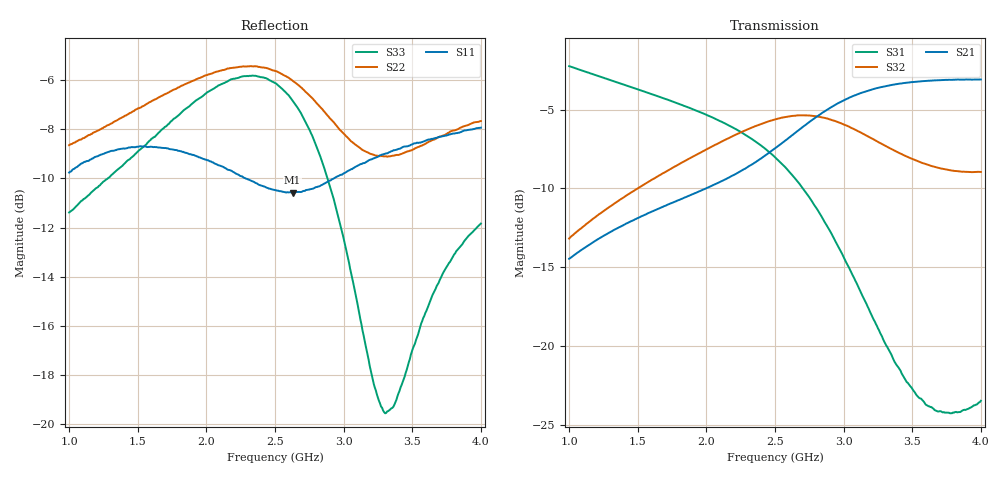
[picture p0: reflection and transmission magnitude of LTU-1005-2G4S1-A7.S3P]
!Agilent Technologies,E5071C,MY46104616,A.09.54
!Date: Mon Mar 28 16:57:22 2011
!Data & Calibration Information:
!Freq	S11:SOLT3(ON)	S12:SOLT3(ON)	S13:SOLT3(ON)
!	S21:SOLT3(ON)	S22:SOLT3(ON)	S23:SOLT3(ON)
!	S31:SOLT3(ON)	S32:SOLT3(ON)	S33:SOLT3(ON)
# Hz S dB R 50
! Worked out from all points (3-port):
!   401 points, 1 GHz to 4 GHz, reference 50 ohm
!   strongest paths, dB at 1 GHz, 1.75 GHz, 2.5 GHz, 3.25 GHz, 4 GHz:
!     S21: -14.5, -10.9, -7.5, -3.6, -3.1
!     S32: -13.2, -8.7, -5.6, -7.0, -9.0
!     S31: -2.2, -4.5, -8.0, -18.9, -23.5
!   lowest |S11| = -10.6 dB at 2.627 GHz (marker M1), VSWR 1.84, Z = 27.2 + j1.98 ohm
!   |S11| at or under -10 dB: 2.286 GHz to 2.929 GHz (643.1 MHz wide, 24.7 % of centre)
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1e9  -9.76 -148.9  -14.47 57.6  -2.24 -54.4
     -14.47 57.7  -8.65 114.4  -13.19 47.3
     -2.24 -54.4  -13.19 47.2  -11.38 -179.4
1.4425e9  -8.75 -167.1  -12.14 48.7  -3.54 -75.4
          -12.12 48.6  -7.34 86.8  -10.33 27.9
          -3.54 -75.4  -10.32 27.7  -9.22 131.3
1.915e9  -9.07 -179.9  -10.32 42.8  -5.02 -100.8
         -10.31 42.7  -6.01 58.3  -7.93 2.8
         -5.03 -100.8  -7.93 2.8  -6.87 78.3
2.1925e9  -9.73 175.5  -9.17 41.0  -6.14 -119.4
          -9.18 40.9  -5.50 41.3  -6.69 -15.9
          -6.14 -119.4  -6.68 -15.9  -5.95 47.4
2.5e9  -10.47 173.4  -7.46 38.5  -8.01 -144.8
       -7.47 38.4  -5.63 21.9  -5.63 -42.5
       -8.02 -144.8  -5.63 -42.5  -6.12 10.2
2.6275e9  -10.58 173.6  -6.60 36.2  -9.17 -156.8
          -6.61 36.2  -6.02 14.8  -5.39 -55.6
          -9.18 -156.8  -5.40 -55.4  -6.83 -6.8
2.9275e9  -10.01 170.5  -4.76 26.0  -13.15 174.4
          -4.75 26.0  -7.71 3.7  -5.69 -89.5
          -13.14 174.5  -5.70 -89.5  -10.83 -52.4
3.3025e9  -9.00 157.4  -3.51 9.2  -19.93 149.6
          -3.51 9.1  -9.10 6.6  -7.29 -131.0
          -19.84 149.7  -7.30 -131.0  -19.55 -156.0
3.6175e9  -8.42 144.2  -3.17 -3.9  -24.00 143.6
          -3.17 -4.0  -8.52 8.4  -8.52 -162.1
          -23.84 143.3  -8.52 -162.1  -15.18 121.9
4e9  -7.93 131.4  -3.09 -17.7  -23.68 132.4
     -3.09 -17.7  -7.67 2.6  -8.98 164.9
     -23.49 132.3  -8.96 164.9  -11.84 83.7
